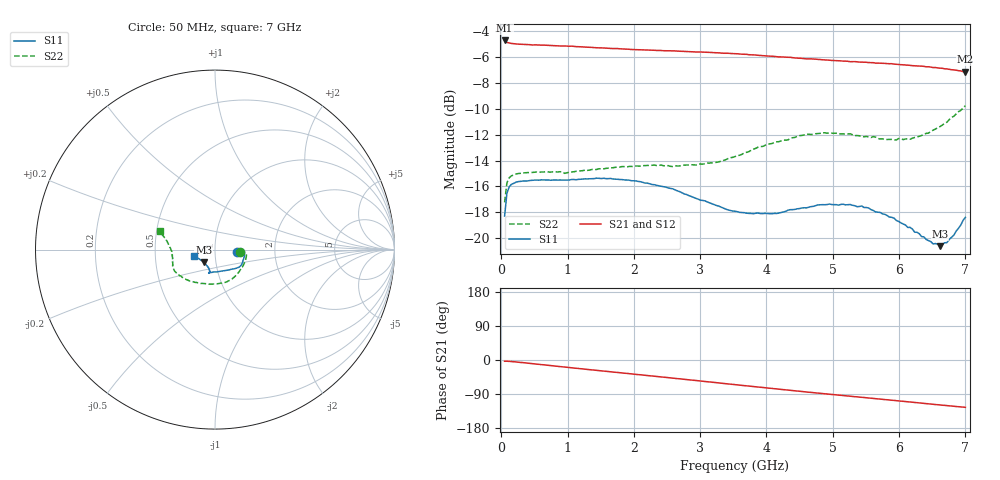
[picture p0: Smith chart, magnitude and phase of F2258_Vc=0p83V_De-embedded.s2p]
! Integrated Device Technology
! Corporate Headquarters
! 6024 Silver Creek Valley Road
! San Jose, CA 95138  USA
! Phone:  1-408-284-8200
! Toll Free:  1-800-223-1366
! Webpage:  http://www.idt.com/
! Timing and RF Division
! 515 Groton Road, Suite 102
! Westford, MA 01886-6024
! Device:  F2258
! Description: Voltage Variable RF Attenuator
! Frequency:  50.0 -  6000.00 MHz
! Package:  3x3 mm Thin QFN Plastic Package: 16 pin
! Ports:  2 RF, 2 DC
!  Pin  1  = NC
!  Pin  2  = NC
!  Pin  3  = RF2  = Port 2
!  Pin  4  = GND
!  Pin  5  = Vdd
!  Pin  6  = NC
!  Pin  7  = VCTRL
!  Pin  8  = NC
!  Pin  9  = GND
!  Pin 10  = RF1  = Port 1
!  Pin 11  = NC
!  Pin 12  = NC
!  Pin 13  = NC
!  Pin 14  = NC
!  Pin 15  = NC
!  Pin 16  = NC
! Vcntrl:  0.830 Volts
! Vdd:  +3.300 Volts
! Current:  1.138 mA
! Data:  The device was measured on a the F2258 evaluation board which has
!  individual transmission lines to the RF pins.  Data was collected
!  using a calibrated network analyzer.  The evaluation board was
!  de-embedded using a TRL calibration technique.
!  The reference plane is the edge of the package pin.
! Misc:  SN 10
!  Action Tracker AT0285
! Date Measured:  2014-12-10
! Date:  2016-01-13  MJV
! Note:
!  Integrated Device Technology supplies this data as a sample of measured
!  data at the package pin for this product.  Your particular data for this
!  product may vary.
!  Data was taken at 25 degrees C.
!  Integrated Device Technology reserves the right to change this data at anytime.
!Freq_(GHz)  S11M_(dB)  S11P_(deg)  S21M_(dB)  S21P_(deg)  S12M_(dB)  S12P_(deg)  S22M_(dB)  S22P_(deg)
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# GHz S dB R 50
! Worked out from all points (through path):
!   201 points, 50 MHz to 7 GHz, reference 50 ohm
!   highest |S21| = -4.71 dB at 50 MHz (marker M1); lowest = -7.1 dB at 7 GHz (marker M2)
!   group delay of S21, straight-line fit = 49.3 ps
!   lowest |S11| = -20.6 dB at 6.618 GHz (marker M3), VSWR 1.21, Z = 43.7 - j6.01 ohm
!   |S11| at or under -10 dB: start of sweep to end of sweep
!   |S22| runs from -17.2 to -9.8 dB; largest |S21 - S12| = 0.0023
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0.05  -18.29 -6.9  -4.71 -3.3  -4.71 -3.3  -17.23 -6.5
0.08475  -16.53 -4.4  -4.86 -3.2  -4.87 -3.2  -15.72 -5.0
0.1195  -16.03 -3.9  -4.91 -3.5  -4.92 -3.5  -15.33 -5.5
0.15425  -15.83 -4.2  -4.94 -4.0  -4.95 -4.0  -15.18 -6.7
0.5365  -15.52 -11.8  -5.05 -10.9  -5.07 -10.9  -14.88 -19.1
0.9535  -15.51 -21.2  -5.14 -18.6  -5.15 -18.6  -14.99 -33.8
1.2315  -15.44 -25.7  -5.22 -23.7  -5.23 -23.7  -14.78 -42.7
1.6485  -15.38 -31.4  -5.33 -31.1  -5.34 -31.1  -14.57 -54.7
2.37825  -15.95 -39.7  -5.48 -44.0  -5.48 -44.0  -14.37 -74.4
2.93425  -16.92 -49.9  -5.60 -54.1  -5.60 -54.1  -14.35 -92.7
3.525  -17.92 -69.5  -5.74 -65.0  -5.75 -65.0  -13.69 -115.9
4.1505  -18.09 -92.9  -5.96 -76.4  -5.99 -76.4  -12.55 -136.9
4.7065  -17.54 -103.7  -6.14 -86.2  -6.16 -86.2  -11.97 -150.0
5.2625  -17.40 -105.2  -6.36 -95.6  -6.34 -95.6  -11.93 -159.2
5.43625  -17.52 -104.2  -6.39 -98.5  -6.37 -98.5  -12.14 -162.0
5.85325  -18.37 -104.3  -6.51 -105.5  -6.51 -105.5  -12.37 -170.5
6.166  -19.17 -108.1  -6.64 -110.8  -6.64 -110.8  -12.35 -177.6
6.5135  -20.45 -124.9  -6.81 -116.8  -6.80 -116.8  -11.65 173.1
6.61775  -20.62 -132.8  -6.85 -118.6  -6.86 -118.6  -11.37 170.3
6.722  -20.35 -141.4  -6.91 -120.4  -6.91 -120.4  -11.03 167.5
6.82625  -19.77 -150.1  -6.99 -122.1  -6.98 -122.1  -10.57 165.5
7  -18.40 -163.8  -7.14 -124.9  -7.14 -125.0  -9.75 161.8
